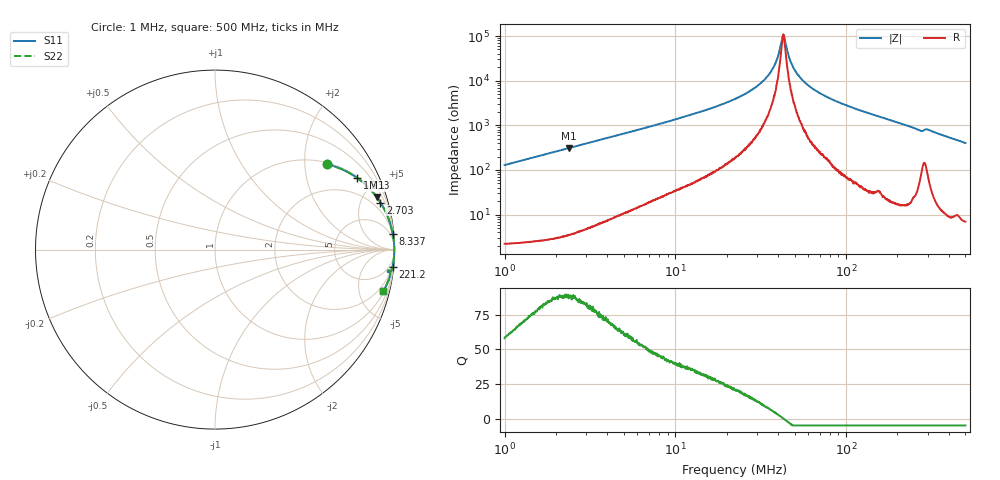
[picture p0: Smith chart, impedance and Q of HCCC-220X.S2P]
!s-Parameter Generated by FASTRON Sdn. Bhd.
!FASTRON P/N : HCCC-220X
!Keysight Technologies,E4991B,MY54100416,A.01.15
!Date: Mon Apr 06 14:31:56 2026
!Version  : Rev00 Mon Apr 06 14:31:56 2026
!Data & Calibration Information:
!PortZ  Port1:50+j0  Port2:50+j0
!When reading, reference impedance value at option line is always used.
! Remarks : This data is being provided solely for informational purposes.
!Freq	S11	S21	S12	S22
# Hz S dB R 50
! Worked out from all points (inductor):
!   1601 points, 1 MHz to 500 MHz, reference 50 ohm
!   read as one part in series: L = 20.5 uH near 1.032 MHz
!   highest Q = 88.3 at 2.369 MHz (marker M1), where L = 20.6 uH
!   self-resonance near 42.77 MHz
!   S11 on the Smith chart (normalised r, x): 1 MHz: 1.04, +2.58; 1.533 MHz: 1.05, +3.96; 2.703 MHz: 1.08, +7.00; 8.337 MHz: 2, +22; 221.2 MHz: 1, -21; 500 MHz: 1.14, -8.03
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1000000  -2.11 37.4  -4.33 -51.6  -4.33 -51.6  -2.11 37.4
1533042  -1.03 26.6  -6.96 -62.6  -6.96 -62.6  -1.03 26.6
2368547  -0.47 18.0  -10.20 -71.3  -10.20 -71.3  -0.47 18.0
2702933  -0.37 15.9  -11.26 -73.4  -11.26 -73.4  -0.37 15.9
2820919  -0.34 15.2  -11.60 -74.1  -11.60 -74.1  -0.34 15.2
7957584  -0.06 5.4  -20.55 -83.4  -20.55 -83.4  -0.06 5.4
8337263  -0.05 5.1  -20.98 -83.6  -20.98 -83.6  -0.05 5.1
2.236068e7  -0.01 1.5  -31.81 -85.8  -31.81 -85.8  -0.01 1.5
2.923332e7  -0.01 0.8  -36.78 -84.9  -36.78 -84.9  -0.01 0.8
3.495212e7  -0.01 0.4  -42.28 -82.1  -42.28 -82.1  -0.01 0.4
3.866622e7  -0.01 0.2  -47.99 -76.1  -47.99 -76.1  -0.01 0.2
4.195229e7  -0.01 0.0  -57.87 -41.9  -57.87 -41.9  -0.01 0.0
4.294146e7  -0.01 -0.0  -60.69 1.3  -60.69 1.3  -0.01 -0.0
4.395396e7  -0.01 -0.1  -57.86 44.8  -57.86 44.8  -0.01 -0.1
4.713694e7  -0.01 -0.2  -49.04 74.9  -49.04 74.9  -0.01 -0.2
4.996481e7  -0.01 -0.3  -44.88 80.5  -44.88 80.5  -0.01 -0.3
5.527421e7  -0.01 -0.5  -40.43 84.2  -40.43 84.2  -0.01 -0.5
6.307767e7  -0.01 -0.8  -36.64 85.9  -36.64 85.9  -0.01 -0.8
9.374216e7  -0.01 -1.8  -29.85 86.7  -29.85 86.7  -0.01 -1.8
1.77937e8  -0.03 -4.3  -22.57 84.9  -22.57 84.9  -0.03 -4.3
2.21172e8  -0.05 -5.6  -20.28 83.5  -20.28 83.5  -0.05 -5.6
5e8  -0.30 -13.9  -12.37 75.1  -12.37 75.1  -0.30 -13.9
